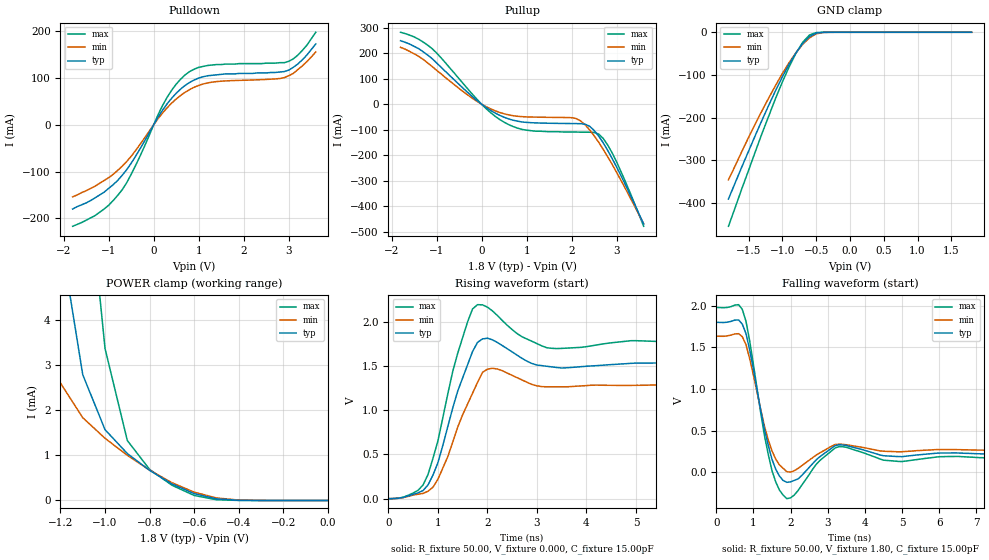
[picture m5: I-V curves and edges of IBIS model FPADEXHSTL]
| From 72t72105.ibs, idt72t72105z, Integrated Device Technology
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|   Model FPADEXHSTL
[Model]   FPADEXHSTL
Model_type   3-state
Polarity   Non-Inverting
Enable   Active-High
Vmeas =  0.900V
C_comp   3.00pF   NA   NA
[Temperature Range]   25.00   85.00   -40.00
[Voltage Range]   1.80V   1.60V   2.00V
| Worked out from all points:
|   slope of the pulldown table from 0 to 0.27 V, typ, clamps not added: 6.57 ohm
|   slope of the pullup table from 0 to 0.27 V, typ, clamps not added: 8.55 ohm
|   GND clamp passes 1 mA (typ) near -0.45 V on its own axis
|   POWER clamp passes 1 mA (typ) near -0.89 V on its own axis
|   rising waveform, R_fixture 50.00, V_fixture 0.000, C_fixture 15.00pF: 20-80 % time 473ps typ, 535ps min, 444ps max; typ from 0 V to 1.52 V
|   falling waveform, R_fixture 50.00, V_fixture 1.80, C_fixture 15.00pF: 20-80 % time 396ps typ, 404ps min, 380ps max; typ from 1.8 V to 0.222 V
[Pulldown]
| voltage   I(typ)   I(min)   I(max)
-1.8V     -180mA     -154mA     -217mA
-1.1V     -144mA     -119mA     -180mA
-700mV    -108mA     -88.57mA   -139mA
-400mV    -66.98mA   -54.66mA   -86.64mA
200mV     31.71mA    25.58mA    41.77mA
400mV     57.04mA    46.47mA    74.01mA
700mV     84.35mA    69.78mA    107mA
1.2V      105mA      89.75mA    127mA
2.7V      112mA      98.23mA    132mA
3V        117mA      105mA      136mA
3.3V      139mA      126mA      159mA
3.6V      173mA      156mA      198mA
[Pullup]
| voltage   I(typ)   I(min)   I(max)
-1.8V     249mA      223mA      282mA
-1.1V     179mA      148mA      218mA
-100mV    14.11mA    10.85mA    18.81mA
500mV     -51.24mA   -37.65mA   -70.6mA
1V        -71.51mA   -49.75mA   -102mA
2V        -75.96mA   -53.01mA   -109mA
2.2V      -76.47mA   -65.7mA    -110mA
2.4V      -86.66mA   -101mA     -110mA
2.6V      -125mA     -149mA     -117mA
2.8V      -181mA     -206mA     -160mA
3.1V      -282mA     -300mA     -266mA
3.6V      -470mA     -469mA     -479mA
[GND_clamp]
| voltage   I(typ)   I(min)   I(max)
-1.8V     -391mA     -346mA     -455mA
-1.5V     -278mA     -246mA     -323mA
-1.3V     -205mA     -183mA     -236mA
-1.1V     -136mA     -124mA     -154mA
-1V       -104mA     -96.2mA    -116mA
-900mV    -74.56mA   -70.77mA   -80.61mA
-800mV    -48.24mA   -47.88mA   -49.04mA
-700mV    -26.16mA   -28.23mA   -23.28mA
-600mV    -10.07mA   -12.98mA   -6.406mA
-500mV    -2.002mA   -3.724mA   -655uA
-400mV    -177uA     -538uA     -28.11uA
1.8V      18.12nA    77.44nA    18nA
[POWER_clamp]
| voltage   I(typ)   I(min)   I(max)
-1.8V     60.33mA    37.96mA    93.88mA
-1.3V     11.23mA    4.427mA    25.79mA
-1.2V     5.851mA    2.598mA    15.98mA
-1.1V     2.782mA    1.831mA    8.297mA
-1V       1.566mA    1.375mA    3.362mA
-900mV    1.038mA    999uA      1.326mA
-800mV    666uA      671uA      687uA
-700mV    367uA      394uA      337uA
-600mV    151uA      184uA      111uA
-500mV    35.57uA    56.06uA    16.17uA
-400mV    4.038uA    9.226uA    1.082uA
0V        18.12nA    21.07nA    20nA
[Ramp]
| variable   typ   min   max
dV/dt_r   0.92/0.29n   0.78/0.34n   1.07/0.26n
dV/dt_f   0.96/0.18n   0.83/0.19n   1.10/0.17n
R_load = 50.00
[Rising Waveform]
R_fixture = 50.00
V_fixture = 0.000
C_fixture = 15.00pF
R_dut = 0.75
L_dut = 8.10nH
C_dut = 0.53pF
| time   V(typ)   V(min)   V(max)
0s        0V         0V         0V
600ps     65.94mV    50.35mV    94.5mV
800ps     155mV      84.15mV    272mV
1ns       406mV      219mV      652mV
1.4ns     1.215V     809mV      1.643V
1.7ns     1.663V     1.192V     2.144V
1.8ns     1.766V     1.313V     2.192V
2.1ns     1.795V     1.473V     2.122V
3.3ns     1.489V     1.264V     1.699V
9.9ns     1.519V     1.283V     1.759V
[Falling Waveform]
R_fixture = 50.00
V_fixture = 1.80
C_fixture = 15.00pF
R_dut = 0.75
L_dut = 8.10nH
C_dut = 0.53pF
| time   V(typ)   V(min)   V(max)
0s        1.8V       1.634V     1.977V
700ps     1.778V     1.627V     1.955V
900ps     1.467V     1.362V     1.575V
1.3ns     509mV      548mV      434mV
1.5ns     156mV      258mV      20.56mV
1.7ns     -43.57mV   90.3mV     -212mV
1.9ns     -119mV     8.792mV    -315mV
3.3ns     331mV      338mV      309mV
4.9ns     190mV      247mV      132mV
9.9ns     222mV      267mV      176mV
